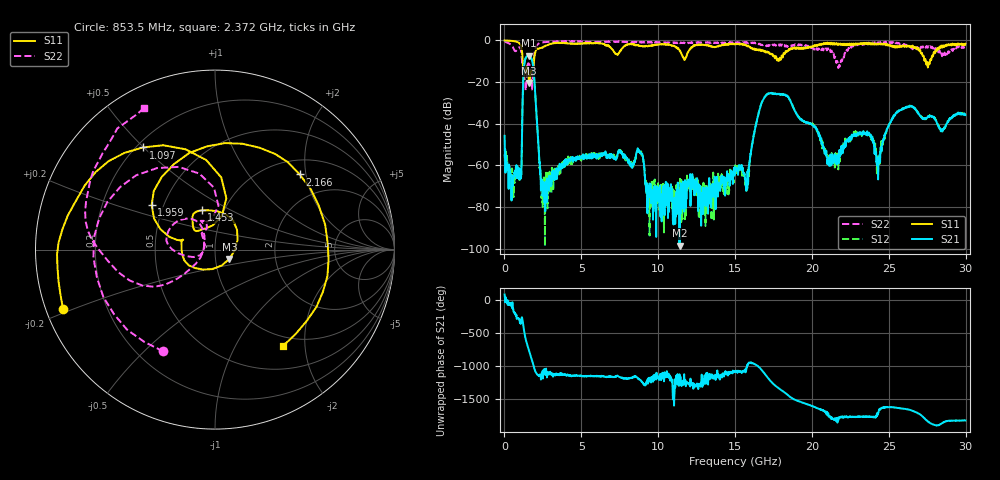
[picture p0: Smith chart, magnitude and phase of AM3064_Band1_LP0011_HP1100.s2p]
# Hz S DB R 50.0
!freq dBS11 angS11 dBS21 angS21 dBS12 angS12 dBS22 angS22
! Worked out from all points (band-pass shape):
!   1600 points, 10 MHz to 29.98 GHz, reference 50 ohm
!   highest |S21| = -7.39 dB at 1.584 GHz (marker M1); lowest = -98.5 dB at 11.39 GHz (marker M2)
!   |S21| within 3 dB of the highest: 1.314 GHz to 1.818 GHz (504.6 MHz wide, 32.2 % of centre)
!   lowest |S11| = -20.4 dB at 1.603 GHz (marker M3), VSWR 1.21, Z = 58.4 - j6.09 ohm
!   |S11| at or under -10 dB: 1.186 GHz to 1.92 GHz (733.5 MHz wide, 47.2 % of centre); 27.4 GHz to 27.68 GHz (282.6 MHz wide, 1.03 % of centre)
!   |S22| runs from -24.1 to -0.3 dB; largest |S21 - S12| = 0.0047
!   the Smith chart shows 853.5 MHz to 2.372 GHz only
!   S11 on the Smith chart (normalised r, x): 853.5 MHz: 0.05, -0.19; 1.097 GHz: 0.23, +0.50; 1.453 GHz: 0.79, +0.36; 1.959 GHz: 0.43, +0.26; 2.166 GHz: 1.33, +1.84; 2.372 GHz: 0.85, -1.60
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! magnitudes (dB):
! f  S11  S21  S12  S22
! 10 MHz  -0.1  -45.8  -54.8  -0.3
! 853.5 MHz  -0.8  -66.1  -61.3  -3.9
! 1.097 GHz  -3.1  -62.8  -64.6  -6.0
! 1.453 GHz  -12.7  -7.7  -7.6  -15.5
! 1.584 GHz  -19.2  -7.4  -7.4  -11.2
! 1.603 GHz  -20.4  -7.4  -7.4  -11.4
! 1.959 GHz  -7.3  -20.7  -20.6  -5.9
! 2.166 GHz  -4.0  -45.5  -44.9  -1.9
! 2.372 GHz  -3.6  -72.0  -68.4  -1.1
! 5.015 GHz  -1.5  -55.5  -55.6  -0.7
! 8.763 GHz  -2.6  -52.8  -53.5  -1.1
! 10 GHz  -2.0  -71.5  -70.9  -0.9
! 11.39 GHz  -4.9  -98.5  -71.4  -1.3
! 15 GHz  -1.9  -62.5  -60.0  -1.3
! 15.77 GHz  -2.6  -68.7  -67.4  -1.0
! 17.14 GHz  -5.8  -25.5  -25.6  -2.7
! 19.99 GHz  -3.2  -40.2  -40.4  -3.4
! 21.15 GHz  -1.5  -58.1  -58.4  -4.3
! 23.33 GHz  -1.6  -44.8  -44.5  -1.6
! 24.34 GHz  -1.9  -57.1  -59.5  -1.2
! 25 GHz  -2.0  -40.7  -40.5  -1.1
! 29.98 GHz  -1.7  -35.9  -35.6  -3.3
